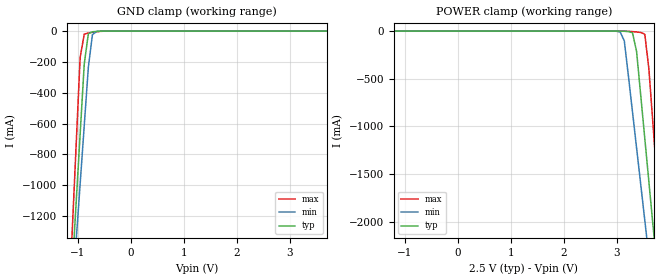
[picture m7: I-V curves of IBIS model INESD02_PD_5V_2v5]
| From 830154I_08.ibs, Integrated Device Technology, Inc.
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| 2.50909e+00   -7.75046e-03   -4.78655e-01   -1.54190e-03
| 2.56364e+00   -1.61412e-02   -1.01365e+00   -3.66568e-03
| 2.61818e+00   -5.97690e-02   -1.54895e+00   -6.99531e-03
| 2.67273e+00   -3.85796e-01   -2.08450e+00   -1.13565e-02
| 2.72727e+00   -1.02854e+00   -2.62029e+00   -1.72285e-02
| 2.78182e+00   -1.67156e+00   -3.15627e+00   -3.57154e-02
| 2.83636e+00   -2.31484e+00   -3.69241e+00   -2.37462e-01
| 2.89091e+00   -2.95829e+00   -4.22868e+00   -1.04190e+00
| 2.94545e+00   -3.60190e+00   -4.76506e+00   -1.86380e+00
| 3.00000e+00   -4.24564e+00   -5.30154e+00   -2.68587e+00
| 3.05455e+00   -4.88948e+00   -5.83811e+00   -3.50806e+00
| 3.10909e+00   -5.53340e+00   -6.37476e+00   -4.33035e+00
| 3.16364e+00   -6.17740e+00   -6.91146e+00   -5.15271e+00
| 3.21818e+00   -6.82145e+00   -7.44822e+00   -5.97513e+00
| 3.27273e+00   -7.46555e+00   -7.98503e+00   -6.79759e+00
| 3.32727e+00   -8.10970e+00   -8.52188e+00   -7.62008e+00
| 3.38182e+00   -8.75387e+00   -9.05876e+00   -8.44259e+00
| 3.43636e+00   -9.39807e+00   -9.59567e+00   -9.26512e+00
| 3.49091e+00   -1.00423e+01   -1.01326e+01   -1.00877e+01
| 3.54545e+00   -1.06865e+01   -1.06696e+01   -1.09102e+01
| 3.60000e+00   -1.13308e+01   -1.12065e+01   -1.17327e+01
[Model] INESD02_PD_5V_2v5
Model_type   Input
Polarity   Non-Inverting
Vinl = .87V
Vinh = 1.62V
|   typ   min   max
C_comp   2pF   1.5pF   2.5pF
|   typ   min   max
[Voltage range]   2.5V   2.375V   2.625V
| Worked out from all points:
|   GND clamp passes 1 mA (typ) near -0.59 V on its own axis
[GND_clamp]
|Voltage   I(typ)   I(min)   I(max)
-2.191V   -7.973A    -7.07A     -9.504A
-1.108V   -1.581A    -1.751A    -1.338A
-1.031V   -1.125A    -1.371A    -755.2mA
-953.6mV  -669.5mA   -992.5mA   -172.1mA
-876.3mV  -213.9mA   -613.7mA   -19.96mA
-799mV    -17.31mA   -235.3mA   -12.11mA
-721.6mV  -4.455mA   -23.01mA   -7.724mA
-644.3mV  -1.863mA   -2.522mA   -4.06mA
5V        97.41uA    121.8uA    75.48uA
[POWER_clamp]
|Voltage   I(typ)   I(min)   I(max)
-2.5V     97.41uA    118.8uA    77.37uA
2.835V    -9.233uA   -44.7uA    -3.208uA
3.067V    -617.5uA   -9.489mA   -116.3uA
3.144V    -1.863mA   -101.8mA   -642.8uA
3.299V    -17.31mA   -847.2mA   -5.362mA
3.376V    -213.9mA   -1.226A    -9.326mA
3.531V    -1.125A    -1.985A    -32.65mA
3.608V    -1.581A    -2.364A    -395.6mA
3.686V    -2.038A    -2.744A    -978.8mA
3.763V    -2.494A    -3.124A    -1.562A
3.84V     -2.95A     -3.503A    -2.145A
4.845V    -8.886A    -8.445A    -9.728A
